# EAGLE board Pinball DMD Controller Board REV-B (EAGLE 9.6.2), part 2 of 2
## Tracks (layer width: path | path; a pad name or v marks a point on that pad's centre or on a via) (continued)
P1 (continued)
  Bottom 0.406: R10.2 211.02,110.63 212.2,111.81 212.2,117.32 216.93,122.05 7B.5 217.32,121.65 219.69,119.29 219.69,94.88 219.29,94.49 | 219.29,94.49 217.32,96.46 7C.1 | 219.29,94.49 219.29,90.94 217.32,88.98 7C.4
P2
  Top 0.406: R9.2 149.61,49.61 143.7,49.61 3D.11 143.31,49.61 141.34,49.61 141.34,53.15 137.79,56.69 136.61,56.69 136.22,57.09 3D.3
PWM  (via drill 0.35)
  Top 0.406: v117.32,112.2 v98.82,112.2 | v117.32,72.83 120.87,69.29 146.06,69.29 147.24,68.11 168.11,68.11 168.9,68.9 v178.74,68.9 | v181.5,36.22 181.89,36.61 v222.83,36.61
  Bottom 0.406: 222.83,50 224.41,48.42 7D.9 | 222.83,50 222.83,56.69 224.41,58.27 7D.13 | v98.82,112.2 98.42,112.6 98.42,134.25 98.82,134.65 98.82,150.79 102.76,154.72 1A.9 | v117.32,112.2 117.72,111.81 117.72,73.23 v117.32,72.83 | v178.74,68.9 179.13,68.5 179.13,46.46 181.5,44.09 v181.5,36.22 | 222.83,50 v222.83,36.61
PWMCOUNTERA  (via drill 0.35)
  Top 0.406: 5E.1 176.77,25.2 179.13,25.2 183.86,20.47 5E.12 190.47,26.64 211.36,26.64 211.41,26.6 218.94,26.6 219.68,27.34 220.48,27.34 221.15,26.67 v222.25,26.67 | v221.62,54.61 221.62,64.77 222.68,65.84 222.68,69.65 v222.88,69.85 | v221.62,87.63 207.01,87.63 205.72,88.92 203.29,88.92 202.56,89.65 202.56,92.08 v201.29,93.34 | v205.74,93.98 211.46,99.69 v216.53,99.69 | v217.81,102.87 v222.88,102.87 | v222.88,113.67 222.88,117.47 7B.9
  Bottom 0.406: v222.25,26.67 221.62,27.3 v221.62,54.61 | v222.88,69.85 222.88,86.36 v221.62,87.63 | v201.29,93.34 201.93,93.98 v205.74,93.98 | v216.53,99.69 216.53,101.6 v217.81,102.87 | v222.88,102.87 222.25,103.5 222.25,113.03 v222.88,113.67
PWMCOUNTERB  (via drill 0.35)
  Top 0.406: 5E.9 184.25,12.99 185.04,13.78 195.28,13.78 196.46,14.96 196.85,14.96 6E.5 196.85,15.35 199.21,17.72 204.33,17.72 6E.11 | v202.36,37.8 231.5,37.8 232.28,38.58 232.28,41.34 v226.77,41.34 | v226.77,64.17 226.77,84.64 231.1,88.98 231.1,94.88 v226.77,94.88 | v218.5,109.84 v226.77,109.84 | v218.5,115.35 222.83,119.69 222.83,121.65 224.41,121.65 7B.10
  Bottom 0.406: 6E.11 204.72,18.11 206.69,20.08 206.69,20.87 204.72,22.84 6E.13 204.33,23.23 203.54,24.02 202.36,24.02 v202.36,37.8 | v226.77,64.17 v226.77,41.34 | v226.77,109.84 v226.77,94.88 | v218.5,115.35 v218.5,109.84
PWMCOUNTERC  (via drill 0.35)
  Top 0.406: v186.61,17.72 196.85,17.72 6E.4 196.85,17.79 198.13,19.07 212.78,19.07 v220.08,26.38 | v134.65,148.43 131.89,148.43 126.38,153.94 124.02,153.94 123.23,154.72 2A.9 | v134.65,139.37 135.83,138.19 159.06,138.19 162.6,134.65 195.67,134.65 197.24,136.22 v229.92,136.22 | v226.77,92.52 v229.92,92.52 | v229.92,127.17 224.8,127.17 7B.12
  Bottom 0.406: v186.61,17.72 186.61,12.6 184.25,10.24 5E.8 | v134.65,139.37 v134.65,148.43 | v229.92,92.52 v229.92,127.17 v229.92,136.22 | v226.77,92.52 226.77,65.75 222.83,61.81 222.83,57.87 220.08,55.12 v220.08,26.38
PWMCOUNTERD  (via drill 0.35)
  Top 0.406: 5E.11 184.25,18.11 185.04,18.9 186.22,18.9 192.52,25.2 196.85,25.2 6E.1 | v88.19,168.9 104.33,168.9 106.3,166.93 111.02,166.93 115.35,162.6 2A.3 | v97.24,90.16 v88.19,90.16 | v95.28,30.32 95.67,30.71 132.68,30.71 133.07,31.1 176.77,31.1 178.35,32.68 v196.85,32.68 | 7B.13 220.87,133.46 v201.18,133.46 | v201.18,110.24 162.99,110.24 162.2,109.45 154.72,109.45 153.54,108.27 v144.09,108.27 | v131.1,111.81 v144.09,111.81 | v131.1,108.27 129.13,106.3 103.15,106.3 101.97,105.12 v88.19,105.12
  Bottom 0.406: v88.19,90.16 v88.19,105.12 v88.19,168.9 | v97.24,90.16 97.24,35.04 95.28,33.07 v95.28,30.32 | 6E.1 v196.85,32.68 | v201.18,110.24 v201.18,133.46 | v144.09,111.81 v144.09,108.27 | v131.1,108.27 v131.1,111.81
PWMSET
  Top 0.406: 6C.9 204.72,79.92 213.38,71.26 218.75,71.26 219.24,71.75 224.79,71.75 224.79,66.04 222.83,64.08 222.83,55.91 224.41,55.91 7D.12
RESET
  Bottom 0.406: S1.4 85.04,127.56 85.04,121.26 S1.3 84.64,120.87 84.64,84.64 B1.RESET
RESETPWM  (via drill 0.35)
  Top 0.406: v232.28,108.27 232.28,112.99 231.5,113.78 227.56,113.78 224.8,116.53 7B.8 | v232.28,46.06 224.8,46.06 7D.8
  Bottom 0.406: v232.28,46.06 v232.28,108.27
ROWCLOCK  (via drill 0.35)
  Top 0.406: v148.82,170.08 164.17,170.08 166.53,167.72 170.08,167.72 176.38,161.42 5A.4 | v127.56,164.57 v133.86,164.57 | v121.26,166.53 118.9,168.9 111.02,168.9 109.84,167.72 106.69,167.72 104.33,170.08 v24.8,170.08 | v24.8,89.37 24.8,86.61 14.17,75.98 9.05,75.98 8.27,75.2 8.27,52.36 9.84,52.36 J3.5
  Bottom 0.406: v148.82,170.08 144.88,170.08 144.49,170.47 133.86,170.47 v133.86,164.57 | v127.56,164.57 127.56,151.18 126.38,150 121.26,150 v121.26,166.53 | v24.8,89.37 v24.8,170.08
ROWDATA  (via drill 0.35)
  Top 0.406: v223.23,123.23 220.47,120.47 218.11,120.47 217.32,119.69 7B.6 | v227.16,28.35 226.77,28.74 207.09,28.74 206.69,28.35 173.62,28.35 171.65,30.32 133.46,30.32 131.5,28.35 107.48,28.35 107.09,27.95 v86.61,27.95 | v17.32,9.05 v86.61,9.05
  Bottom 0.406: v223.23,123.23 222.83,122.83 222.83,115.35 227.95,110.24 227.95,30.32 227.16,29.53 v227.16,28.35 | v86.61,9.05 v86.61,27.95 | v17.32,9.05 14.17,12.21 14.17,57.87 13.39,58.66 8.66,58.66 8.66,55.91 9.84,54.72 J3.3
RX
  Top 0.406: R6.1 27.95,51.97 28.74,51.18 32.68,51.18 B1.0
RX2  (via drill 0.35)
  Top 0.406: v36.61,126.38 27.95,135.04 11.81,135.04 X1.3
  Bottom 0.406: v36.61,126.38 37.01,125.98 37.01,42.13 33.07,38.19 B1.17
SD_CS  (via drill 0.35)
  Top 0.406: v79.13,20.87 78.35,20.87 78.35,17.72 76.77,16.14 75.59,16.14 74.02,17.72 B1.53
  Bottom 0.406: J2.8 57.87,144.09 57.87,141.73 J2.7 57.87,141.34 61.42,137.79 61.42,46.85 77.56,30.71 77.56,25.59 78.74,24.41 78.74,21.26 v79.13,20.87
SD_FAIL
  Bottom 0.406: R8.1 35.43,154.72 35.43,100.79 36.22,100 36.22,86.22 33.07,83.07 B1.12
SD_MISO
  Bottom 0.406: J2.14 50.39,144.09 50.39,141.73 J2.13 50.39,141.34 53.94,137.79 53.94,51.58 53.54,51.18 J1.1
SD_MOSI  (via drill 0.35)
  Top 0.406: v60.24,48.42 60.24,48.03 59.05,46.85 57.09,46.85 55.91,48.03 J1.4
  Bottom 0.406: J2.10 55.51,144.09 55.51,141.73 J2.9 59.84,137.01 59.84,48.82 v60.24,48.42
SD_SCK
  Bottom 0.406: J2.12 52.76,144.09 52.76,141.73 J2.11 52.76,141.34 54.72,139.37 54.72,51.97 55.51,51.18 J1.3
SERIALDATA  (via drill 0.35)
  Top 0.406: v190.55,82.28 196.85,82.28 6C.7 | v190.55,133.46 171.26,133.46 167.32,129.53 162.6,129.53 158.27,133.86 158.27,137.4 135.83,137.4 134.65,136.22 v100,136.22 | v66.14,113.39 v99.61,113.39 | v66.14,45.28 35.83,45.28 33.86,47.24 32.28,47.24 29.53,44.49 29.53,40.55 9.45,40.55 8.66,41.34 8.66,44.09 9.84,44.09 J3.11
  Bottom 0.406: v190.55,133.46 v190.55,82.28 | v100,136.22 99.61,135.83 99.61,134.25 99.21,133.86 99.21,113.78 v99.61,113.39 | v66.14,45.28 v66.14,113.39
TX
  Top 0.406: R5.1 25.59,55.51 27.56,53.54 32.68,53.54 B1.1
TX2  (via drill 0.35)
  Top 0.406: v31.5,86.61 27.56,90.55 v14.57,90.55
  Bottom 0.406: v31.5,86.61 31.5,42.13 32.68,40.95 B1.16 | v14.57,90.55 14.57,128.35 11.81,131.1 X1.4
VCC  (via drill 0.35)
  Top 1.016: 110.49,3.81 109.22,5.08 v109.22,8.89 | 147.32,173.99 v147.32,168.91 | 167.64,173.99 v167.64,168.91 | 187.96,173.99 v187.96,168.91 | 208.28,173.99 v208.28,168.91 | 110.49,173.99 109.22,172.72 v109.22,168.91 | 208.28,3.81 v208.28,8.89 | 187.96,3.81 v187.96,8.89 | 167.64,3.81 v167.64,8.89 | 147.32,3.81 v147.32,8.89 | R4.1 22.86,158.75 3.81,158.75 | 2A.14 123.19,173.99 | 4A.5 v147.32,157.48 | v187.96,121.92 6B.5 | 5E.5 v167.64,15.24 | 7B.14 237.49,132.08 | C9.1 237.49,106.68 | 7C.14 237.49,96.52 | 7D.14 237.49,60.96
  Top 2.54: X1.2 4.22,139.29 3.81,139.7 | X2.2 11.43,83.82 X2.1
  Top 5.08: 3.81,83.82 3.81,17.78 17.78,3.81 110.49,3.81 147.32,3.81 167.64,3.81 187.96,3.81 208.28,3.81 226.06,3.81 237.49,15.24 237.49,60.96 237.49,96.52 237.49,106.68 237.49,132.08 237.49,162.56 226.06,173.99 208.28,173.99 187.96,173.99 167.64,173.99 147.32,173.99 123.19,173.99 110.49,173.99 17.78,173.99 3.81,160.02 3.81,158.75 3.81,139.7 3.81,83.82 | 11.43,83.82 3.81,83.82
  Bottom 1.016: v109.22,168.91 109.22,167.64 | 109.22,167.64 109.22,132.08 | 109.22,132.08 109.22,121.92 | 109.22,121.92 109.22,106.68 | 109.22,106.68 109.22,96.52 | 109.22,96.52 109.22,86.36 | 109.22,86.36 109.22,71.12 | 109.22,71.12 109.22,60.96 | 109.22,60.96 109.22,50.8 | 109.22,50.8 109.22,25.4 | 109.22,25.4 109.22,15.24 | 109.22,15.24 v109.22,8.89 | 147.32,133.35 v147.32,157.48 v147.32,168.91 3A.16 | 147.32,133.35 147.32,106.68 | 147.32,106.68 147.32,97.79 | 147.32,97.79 147.32,62.23 | 147.32,62.23 147.32,41.91 | 147.32,41.91 v147.32,8.89 | v167.64,168.91 167.64,135.89 | 167.64,135.89 167.64,97.79 | 167.64,97.79 167.64,71.12 | 167.64,71.12 167.64,62.23 | 167.64,62.23 167.64,26.67 | 167.64,26.67 v167.64,15.24 v167.64,8.89 | 187.96,132.08 v187.96,168.91 5A.16 | 187.96,132.08 v187.96,121.92 187.96,106.68 | 187.96,106.68 187.96,97.79 | 187.96,97.79 187.96,64.77 | 187.96,64.77 v187.96,8.89 | v208.28,168.91 208.28,167.64 | 208.28,167.64 208.28,102.87 | 208.28,102.87 208.28,97.79 | 208.28,97.79 208.28,71.12 | 208.28,71.12 208.28,60.96 | 208.28,60.96 208.28,25.4 | 208.28,25.4 v208.28,8.89 | C4.1 109.22,71.12 | C3.1 109.22,106.68 | C5.1 147.32,106.68 | C6.1 167.64,71.12 | C7.1 187.96,106.68 | C8.1 208.28,71.12 | 208.28,102.87 R10.1 | 147.32,41.91 R9.1 | 1E.14 109.22,25.4 | 109.22,15.24 2E.5 | 1D.14 109.22,60.96 | 109.22,50.8 2D.5 | 1C.14 109.22,96.52 | 109.22,86.36 2C.5 | 1B.14 109.22,132.08 | 109.22,121.92 2B.5 | 1A.14 109.22,167.64 | 3C.16 147.32,97.79 | 3B.16 147.32,133.35 | 3D.16 147.32,62.23 | 4E.16 167.64,26.67 | 4D.16 167.64,62.23 | 4C.16 167.64,97.79 | 4B.20 167.64,135.89 | 5B.14 187.96,132.08 | 5C.16 187.96,97.79 | 5D.20 187.96,64.77 | 6E.14 208.28,25.4 | 6D.14 208.28,60.96 | 6C.16 208.28,97.79
  Bottom 1.016: 6A.14 208.28,167.64
WEA  (via drill 0.35)
  Top 0.406: v138.98,72.83 139.37,73.23 156.69,73.23 v157.09,73.62 | v166.14,76.77 v157.09,76.77 | v166.14,96.46 166.14,99.21 v164.17,99.21
  Bottom 0.406: v138.98,72.83 138.98,57.48 136.22,54.72 3D.4 | v157.09,76.77 v157.09,73.62 | v166.14,76.77 166.53,77.17 166.53,96.06 v166.14,96.46 | v164.17,99.21 164.17,112.99 4B.11
WEB  (via drill 0.35)
  Top 0.406: v180.71,26.38 180.31,26.77 166.53,26.77 165.35,27.95 v144.09,27.95
  Bottom 0.406: v180.71,26.38 180.71,30.71 182.68,32.68 182.68,40.55 183.86,41.73 5D.11 | v144.09,27.95 143.7,28.35 143.7,44.09 3D.9
WHICHBUFFER
  Top 0.406: 1E.9 102.76,12.99 101.97,13.78 99.21,13.78 96.46,16.54 84.25,16.54 82.68,14.96 74.02,14.96 71.26,17.72 B1.51
WRITE
  Top 0.406: 1E.5 94.88,14.96 94.09,14.17 72.44,14.17 68.9,17.72 B1.49

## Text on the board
tPlace: +12 | +5 | SD Failure | A | Board and Design are Licensed under the / Creative Commons License CC BY-SA 4.0 | Graphics | https://creativecommons.org/licenses/by-sa/4.0/ | Kincaid Arcade / DMD Controller | REV-B | Designed By: / Alexander K. Haley / (A 17 year old!) | Reset | KincaidArcade.com | B | (c) Kincaid Arcade / 6/24/2021 | The REV-B board was finished as an 18 year old / as I only just got around to incorporating the / wire mods I made to REV-A to get it working. | C | D | 1 | 2 | 3 | 4 | 5 | 6 | 7 | E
